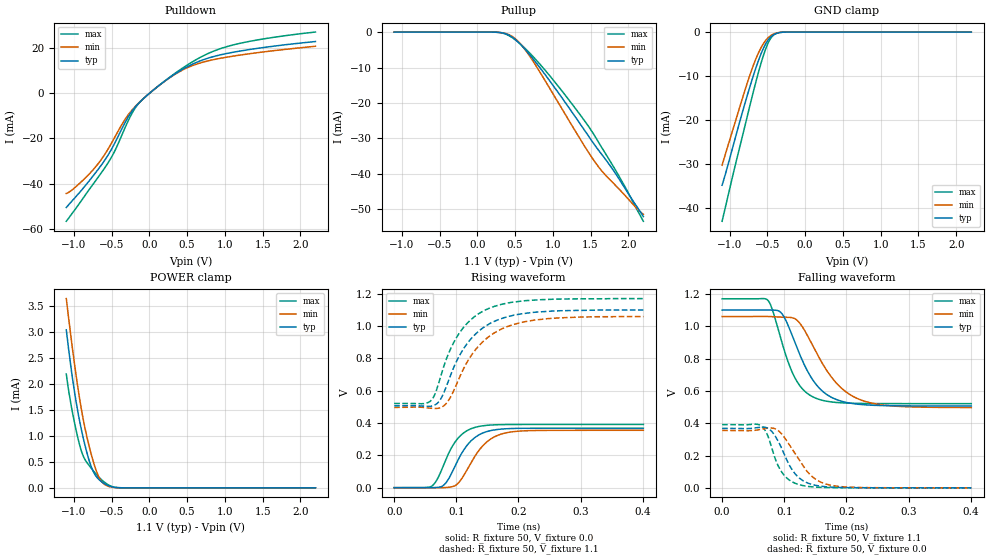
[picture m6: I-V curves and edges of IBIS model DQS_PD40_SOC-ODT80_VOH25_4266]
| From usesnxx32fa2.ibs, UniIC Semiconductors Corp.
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| DQS_PD40_SOC-ODT80_VOH25_4266
| (40 Ohm Pulldown, 80 Ohm System ODT Setting, VOH=VDDQ/2.5, 3200-4266Mbps)
[Model]   DQS_PD40_SOC-ODT80_VOH25_4266
Model_type   I/O
Vinl = 160.000mV
Vinh = 280.000mV
Vmeas = 220.000mV
Vref = 0.0mV
Cref = 0.0pF
Rref = 80.000Ohm
|   typ   min   max
|C_comp   0.849pF   0.799pF   0.899pF
C_comp_pullup   0.4245pF   0.3995pF   0.4495pF
C_comp_pulldown   0.4245pF   0.3995pF   0.4495pF
| Note: C_comp changes when the ODT circuit is enabled.
[Model Spec]
| Input threshold voltage corners
Vinl   0.1600V   0.1520V   0.1740V
Vinh   0.2800V   0.2720V   0.2940V
| Measurement voltage corners
Vmeas   0.2200V   0.2120V   0.2340V
| Timing spec test load voltage corners
Vref   0.0000V   0.0000V   0.0000V
| Dynamic Overshoot Parameters from LPDDR4 Specification
D_overshoot_ampl_h   0.30   NA   NA
D_overshoot_ampl_l   0.30   NA   NA
D_overshoot_area_h   0.1n   NA   NA
D_overshoot_area_l   0.1n   NA   NA
[Voltage Range]   1.1000V   1.0600V   1.1700V
[Pullup Reference]   1.1000V   1.0600V   1.1700V
| Junction Temperature (Ambient temp is 35C typ 95C min -40C max)
[Temperature Range]   50.0   110.0   -40.0
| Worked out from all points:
|   slope of the pulldown table from 0 to 0.165 V, typ, clamps not added: 36.9 ohm
|   slope of the pullup table from 0 to 0.165 V, typ, clamps not added: 17.7 kohm
|   GND clamp passes 1 mA (typ) near -0.45 V on its own axis
|   POWER clamp passes 1 mA (typ) near -0.88 V on its own axis
|   rising waveform, R_fixture 50, V_fixture 0.0: 20-80 % time 34.6ps typ, 38.2ps min, 31.6ps max; typ from 0.001 V to 0.368 V
|   falling waveform, R_fixture 50, V_fixture 1.1: 20-80 % time 45.6ps typ, 57.6ps min, 35.8ps max; typ from 1.1 V to 0.507 V
|   rising waveform, R_fixture 50, V_fixture 1.1: 20-80 % time 56.3ps typ, 59.8ps min, 51.7ps max; typ from 0.507 V to 1.1 V
|   falling waveform, R_fixture 50, V_fixture 0.0: 20-80 % time 31.3ps typ, 39.3ps min, 25.3ps max; typ from 0.368 V to 0.001 V
[Pulldown]
|   Voltage   I(typ)   I(min)   I(max)
-1.1V     -50.64mA   -44.4mA    -56.73mA
-905.3mV  -43.23mA   -39.35mA   -47.84mA
-677.6mV  -33.7mA    -31.18mA   -37.18mA
-486.2mV  -23.86mA   -21.19mA   -27.39mA
-317.9mV  -12.72mA   -11.35mA   -14.94mA
-182.6mV  -5.881mA   -5.661mA   -6.291mA
-63.8mV   -1.901mA   -1.884mA   -1.878mA
229.9mV   6.064mA    5.989mA    6.147mA
573.1mV   12.96mA    12.33mA    14.03mA
959.2mV   17.21mA    15.66mA    20.03mA
1.434V    19.96mA    18.04mA    23.71mA
2.2V      22.98mA    20.89mA    27.18mA
[GND Clamp]
|   Voltage   I(typ)   I(min)   I(max)
-1.1V     -34.75mA   -30.21mA   -42.92mA
-944.9mV  -25.23mA   -21.44mA   -31.56mA
-793.1mV  -15.92mA   -12.96mA   -20.97mA
-720.5mV  -11.75mA   -9.183mA   -15.88mA
-661.1mV  -8.569mA   -6.434mA   -11.86mA
-588.5mV  -5.115mA   -3.68mA    -7.305mA
-519.2mV  -2.566mA   -1.832mA   -3.663mA
-466.4mV  -1.295mA   -942uA     -1.691mA
-413.6mV  -565.1uA   -416.8uA   -621.5uA
-350.9mV  -165.9uA   -125.8uA   -147.9uA
-261.8mV  -17.69uA   -15.38uA   -11.03uA
2.2V      0A         0A         0A
[Pullup]
|   Voltage   I(typ)   I(min)   I(max)
-1.1V     4.106uA    7.431uA    1.361uA
266.2mV   -69.11uA   -66.76uA   -71.72uA
391.6mV   -603.6uA   -501uA     -718.6uA
500.5mV   -2.041mA   -1.829mA   -2.142mA
606.1mV   -4.221mA   -4.208mA   -4.061mA
741.4mV   -7.628mA   -8.301mA   -6.975mA
1.088V    -17.54mA   -20.45mA   -15.71mA
1.458V    -28.85mA   -33.42mA   -26.13mA
1.573V    -32.37mA   -37.08mA   -29.9mA
1.695V    -35.82mA   -40.29mA   -34.18mA
1.946V    -43.74mA   -45.84mA   -43.25mA
2.2V      -52.05mA   -51.4mA    -53.39mA
[POWER Clamp]
|   Voltage   I(typ)   I(min)   I(max)
-1.1V     3.033mA    3.633mA    2.184mA
-1.044V   2.381mA    2.967mA    1.653mA
-968mV    1.637mA    2.139mA    1.094mA
-905.3mV  1.155mA    1.553mA    732.3uA
-849.2mV  799uA      1.125mA    535.5uA
-776.6mV  434.1uA    683.2uA    390.2uA
-707.3mV  225.5uA    345.3uA    267.6uA
-651.2mV  138.6uA    162.4uA    181.2uA
-595.1mV  80.76uA    68.29uA    109.2uA
-486.2mV  16.72uA    10.16uA    20.92uA
-367.4mV  1.19uA     876.5nA    944.1nA
2.2V      0A         0A         0A
[Ramp]
|   typ   min   max
| 20% - 80%
dV/dt_r   220.67m/34.62p   212.99m/38.16p   234.73m/31.58p
dV/dt_f   356.03m/45.65p   337.71m/57.58p   389.19m/35.75p
| 25% - 75%
|dV/dt_r   183.89m/27.56p   177.50m/30.42p   195.60m/25.07p
|dV/dt_f   296.69m/36.41p   281.42m/45.98p   324.32m/28.47p
R_load = 50
[Rising Waveform]
R_fixture = 50
V_fixture = 0.0
|   Time   V(typ)   V(min)   V(max)
0s        576.2uV    460uV      427uV
59ps      302.1uV    60.2uV     6.861mV
68ps      1.699mV    -527.5uV   44.07mV
78ps      11.14mV    298.1uV    126.8mV
103ps     173.9mV    28.19mV    307.8mV
117ps     261.2mV    109.9mV    352.6mV
132ps     316.6mV    207.5mV    375.5mV
156ps     354.2mV    303.3mV    388.2mV
188ps     366.4mV    345.1mV    391.3mV
401ps     368.4mV    355.4mV    391.6mV
[Falling Waveform]
R_fixture   = 50
V_fixture   = 1.1
V_fixture_min = 1.06
V_fixture_max = 1.17
|   Time   V(typ)   V(min)   V(max)
0s        1.1V       1.06V      1.17V
74ps      1.1V       1.06V      1.159V
96ps      1.079V     1.056V     903.5mV
115ps     920.8mV    1.05V      697.3mV
128ps     797.9mV    1.004V     618.1mV
149ps     651.2mV    856.1mV    557.7mV
184ps     546.5mV    648mV      528.4mV
223ps     516mV      544.4mV    522.5mV
279ps     507.9mV    505.4mV    521.5mV
401ps     506.6mV    497.1mV    521.4mV
[Rising Waveform]
R_fixture   = 50
V_fixture   = 1.1
V_fixture_min = 1.06
V_fixture_max = 1.17
|   Time   V(typ)   V(min)   V(max)
0s        506.5mV    496.8mV    521.3mV
57ps      503.2mV    492.6mV    532.3mV
66ps      513.1mV    490.1mV    582.9mV
79ps      579.9mV    504.6mV    741.8mV
94ps      727.7mV    586.1mV    885.4mV
112ps     862.2mV    739.3mV    993.7mV
130ps     947.6mV    849.8mV    1.06V
152ps     1.011V     933.9mV    1.109V
227ps     1.086V     1.038V     1.161V
401ps     1.1V       1.059V     1.17V
[Falling Waveform]
R_fixture = 50
V_fixture = 0.0
|   Time   V(typ)   V(min)   V(max)
0s        368.5mV    355.6mV    391.7mV
58ps      374mV      358.9mV    392.3mV
75ps      365.9mV    370.3mV    307.4mV
86ps      317mV      364.6mV    174.7mV
96ps      243.4mV    333.4mV    97.47mV
111ps     122.2mV    250.2mV    41.27mV
126ps     55.84mV    161.1mV    17.92mV
150ps     16.22mV    54.74mV    5.098mV
181ps     3.876mV    12.57mV    1.335mV
401ps     621.2uV    531.5uV    445.4uV
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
